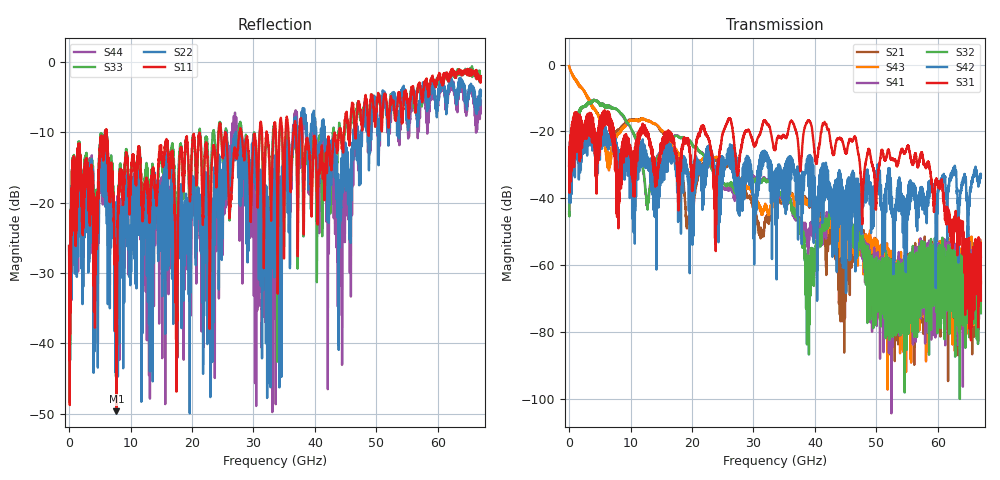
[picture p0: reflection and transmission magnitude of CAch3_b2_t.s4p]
!Agilent Technologies,N5247A,US51170199,A.09.90.13
!Agilent N5247A: A.09.90.13
!Date: Tuesday, October 23, 2018 11:20:56
!Correction: S11(Full 4 Port(1,2,3,4))
!S12(Full 4 Port(1,2,3,4))
!S13(Full 4 Port(1,2,3,4))
!S14(Full 4 Port(1,2,3,4))
!S21(Full 4 Port(1,2,3,4))
!S22(Full 4 Port(1,2,3,4))
!S23(Full 4 Port(1,2,3,4))
!S24(Full 4 Port(1,2,3,4))
!S31(Full 4 Port(1,2,3,4))
!S32(Full 4 Port(1,2,3,4))
!S33(Full 4 Port(1,2,3,4))
!S34(Full 4 Port(1,2,3,4))
!S41(Full 4 Port(1,2,3,4))
!S42(Full 4 Port(1,2,3,4))
!S43(Full 4 Port(1,2,3,4))
!S44(Full 4 Port(1,2,3,4))
!S4P File: Measurements: <S11,S12,S13,S14>,
!<S21,S22,S23,S24>,
!<S31,S32,S33,S34>,
!<S41,S42,S43,S44>:
# Hz S  dB  R 50
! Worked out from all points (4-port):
!   6701 points, 10 MHz to 67 GHz, reference 50 ohm
!   strongest paths, dB at 10 MHz, 16.76 GHz, 33.51 GHz, 50.25 GHz, 67 GHz:
!     S31: -30.3, -22.3, -25.3, -32.8, -70.7
!     S42: -30.3, -26.0, -31.8, -36.7, -32.9
!     S32: -44.2, -22.1, -36.8, -67.8, -74.5
!     S41: -44.6, -21.9, -36.7, -64.4, -65.7
!     S43: -0.5, -24.4, -40.7, -60.8, -65.5
!     S21: -0.5, -25.7, -41.6, -59.2, -57.6
!   lowest |S11| = -49.7 dB at 7.709 GHz (marker M1), VSWR 1.01, Z = 49.8 - j0.275 ohm
!   |S11| at or under -10 dB: start of sweep to 5.859 GHz; 6.066 GHz to 24.34 GHz (18.27 GHz wide, 120 % of centre); 37.89 GHz to 43.98 GHz (6.091 GHz wide, 14.9 % of centre)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
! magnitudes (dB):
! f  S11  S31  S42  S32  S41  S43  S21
! 10 MHz  -26.2  -30.3  -30.3  -44.2  -44.6  -0.5  -0.5
! 7.709 GHz  -49.7  -28.9  -25.2  -13.3  -13.4  -21.6  -20.0
! 12.72 GHz  -17.4  -20.5  -28.5  -41.7  -41.3  -16.9  -16.8
! 19.75 GHz  -18.7  -29.8  -39.8  -22.9  -22.9  -32.3  -48.4
! 23.2 GHz  -14.9  -26.2  -27.4  -31.2  -31.4  -27.2  -27.4
! 55.09 GHz  -5.9  -24.6  -44.3  -58.1  -65.3  -62.8  -72.2
! 67 GHz  -2.0  -70.7  -32.9  -74.5  -65.7  -65.5  -57.6
